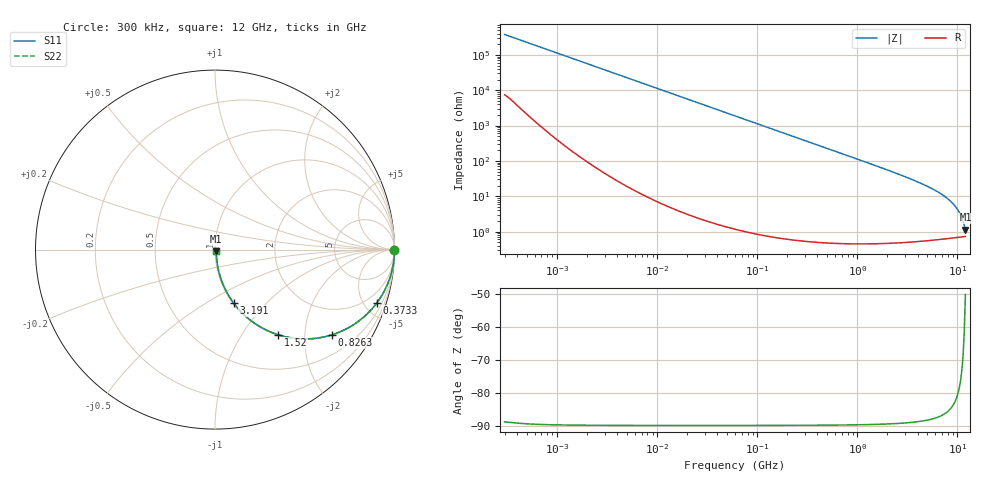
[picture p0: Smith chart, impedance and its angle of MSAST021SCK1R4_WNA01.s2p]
! MSAST021SCK1R4_WNA01  S-PARAMETER MODEL  ( General Type )
! Model Generated by TAIYO YUDEN Corporation (http://www.ty-top.com)
! Version 2.0
! TAIYO YUDEN Control No. 181101
! Copyright(c) 2015 TAIYO YUDEN CO.,LTD. All Rights Reserved.
! Product Description (link to TY-COMPAS)
! https://ds.yuden.co.jp/TYCOMPAS/or/detail?pn=MSAST021SCK1R4BWNA01&u=M
! Products Name : Multilayer Ceramic Capacitors
! Characteristics :
!  Capacitance : 1.4 pF , Rated Voltage : 25V , TCC : CK / C0K
!  Case Size : 0.25 x 0.125 / 0.0098 x 0.0049 [mm/inch] , Thickness : 0.125 / 0.0049 [mm/inch]
!  (Conditions: Temperature = 25 degC , DC Bias Current/Voltage = 0A / 0V)
! External Node Assignments :
!  1  o---| |---o  2
! GND o---------o GND
! Frequency Range : 0.3MHz  -  12000MHz  [ 401 STEP ]
# MHz S RI R 50
! Freq[MHz].  S11 Real  S11 Imag  S21 Real  S21 Imag  S12 Real  S12 Imag  S22 Real  S22 Imag
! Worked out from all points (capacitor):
!   401 points, 300 kHz to 12 GHz, reference 50 ohm
!   read as one part in series: C = 1.4 pF near 316.3 kHz
!   lowest |Z| = 1.14 ohm at 12 GHz (marker M1)
!   S11 on the Smith chart (normalised r, x): 300 kHz: open; 373.3 MHz: 1.01, -6.09; 826.3 MHz: 1.01, -2.74; 1.52 GHz: 1.01, -1.47; 3.191 GHz: 1.01, -0.67; 12 GHz: 1.01, -0.02
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0.3  1 -0.000264  5.23e-06 0.000264  5.23e-06 0.000264  1 -0.000264
1.769972  1 -0.00156  5.32e-06 0.00156  5.32e-06 0.00156  1 -0.00156
10.44266  0.9999 -0.00918  9e-05 0.00918  9e-05 0.00918  0.9999 -0.00918
60  0.9972 -0.0526  0.00281 0.0526  0.00281 0.0526  0.9972 -0.0526
155.7172  0.9815 -0.1344  0.0185 0.1344  0.0185 0.1344  0.9815 -0.1344
244.3004  0.9556 -0.2054  0.0444 0.2054  0.0444 0.2054  0.9556 -0.2054
353.9943  0.9111 -0.2838  0.0889 0.2838  0.0889 0.2838  0.9111 -0.2838
373.2558  0.9021 -0.2963  0.0979 0.2963  0.0979 0.2963  0.9021 -0.2963
555.3718  0.8062 -0.3942  0.1938 0.3942  0.1938 0.3942  0.8062 -0.3942
826.3444  0.6519 -0.4747  0.3481 0.4747  0.3481 0.4747  0.6519 -0.4747
1135.593  0.4965 -0.4977  0.5035 0.4977  0.5035 0.4977  0.4965 -0.4977
1519.776  0.3529 -0.4748  0.6471 0.4748  0.6471 0.4748  0.3529 -0.4748
2088.533  0.2209 -0.4105  0.7791 0.4105  0.7791 0.4105  0.2209 -0.4105
3190.978  0.1036 -0.2974  0.8964 0.2974  0.8964 0.2974  0.1036 -0.2974
5565.855  0.0315 -0.1582  0.9685 0.1582  0.9685 0.1582  0.0315 -0.1582
6879.757  0.019 -0.113  0.981 0.113  0.981 0.113  0.019 -0.113
8064.993  0.0131 -0.0815  0.9869 0.0815  0.9869 0.0815  0.0131 -0.0815
8966.534  0.0104 -0.0614  0.9896 0.0614  0.9896 0.0614  0.0104 -0.0614
9968.853  0.00855 -0.0419  0.9914 0.0419  0.9914 0.0419  0.00855 -0.0419
10793.46  0.00773 -0.0275  0.9923 0.0275  0.9923 0.0275  0.00773 -0.0275
11686.27  0.00735 -0.0133  0.9927 0.0133  0.9927 0.0133  0.00735 -0.0133
12000  0.00731 -0.00861  0.9927 0.00861  0.9927 0.00861  0.00731 -0.00861
